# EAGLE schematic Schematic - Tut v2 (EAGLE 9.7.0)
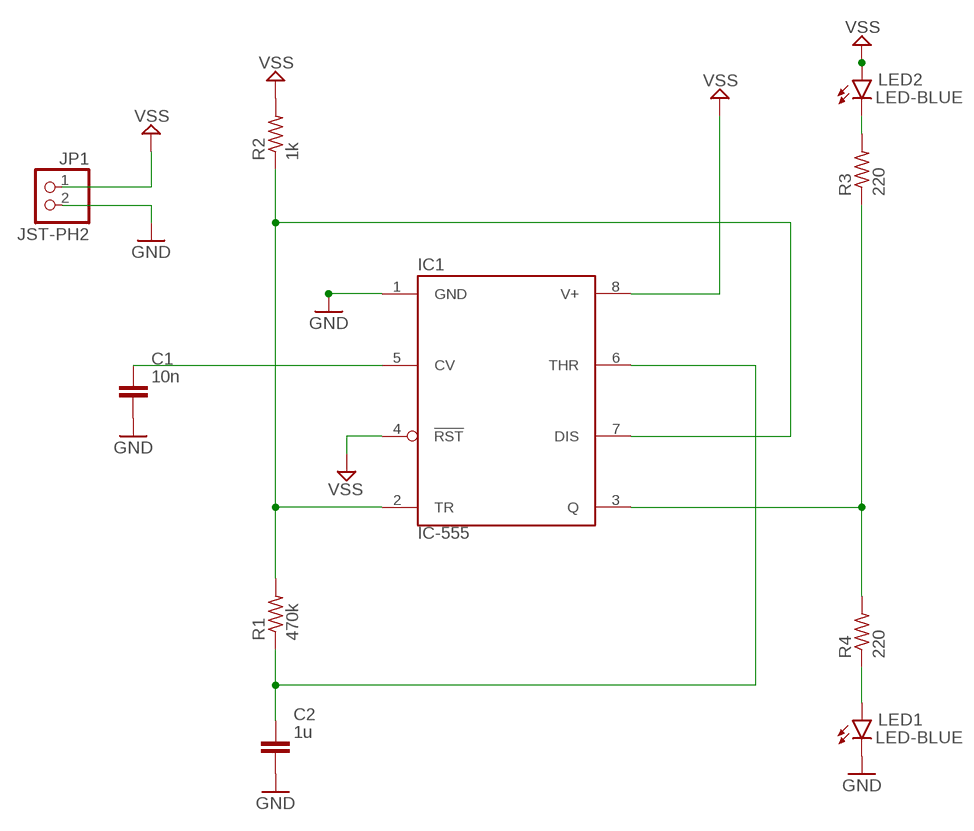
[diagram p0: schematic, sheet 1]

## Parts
C1  10n  C_CHIP-1206(3216-METRIC)  [CAPC3216X135]
C2  1u  C_CHIP-1206(3216-METRIC)  [CAPC3216X135]
IC1  IC-555  LM555NR-PDIP-T8  [P(R-PDIP-T8)]
JP1  JST-PH2  JSTPH2  [JSTPH2]
LED1  LED-BLUE  LED_CHIP_BLUE-2012  [LEDC2012X110N_B]
LED2  LED-BLUE  LED_CHIP_BLUE-2012  [LEDC2012X110N_B]
R1  470k  R-US_CHIP-1206(3216-METRIC)  [RESC3216X70]
R2  1k  R-US_CHIP-1206(3216-METRIC)  [RESC3216X70]
R3  220  R-US_CHIP-1206(3216-METRIC)  [RESC3216X70]
R4  220  R-US_CHIP-1206(3216-METRIC)  [RESC3216X70]

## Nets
GND: C1.2 C2.2 JP1.2 LED1.1(C)
N$1: C1.1 IC1.5(CV)
N$2: IC1.2(TR) IC1.7(DIS) R1.2 R2.1
N$3: C2.1 IC1.6(THR) R1.1
N$4: IC1.3(Q) R3.1 R4.2
N$5: LED2.1(C) R3.2
N$6: LED1.2(A) R4.1
N$8: IC1.1(GND)
VSS: IC1.4(!RST) IC1.8(V+) JP1.1 LED2.2(A) R2.2

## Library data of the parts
C1 C2 = Tutorial - Fusion 360:C: Capacitor - Generic; CATEGORY: Capacitor
IC1 = Tutorial - Fusion 360:LM555N
JP1 = Tutorial - Fusion 360:JSTPH2
LED1 LED2 = Tutorial - Fusion 360:LED_CHIP: LED - Generic; CATEGORY: Opto-Electronic; COLOR: Blue; SUB-CATEGORY: LED
R1-R4 = Tutorial - Fusion 360:R-US: Resistor Fixed - ANSI; CATEGORY: Resistor; SUB-CATEGORY: Fixed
